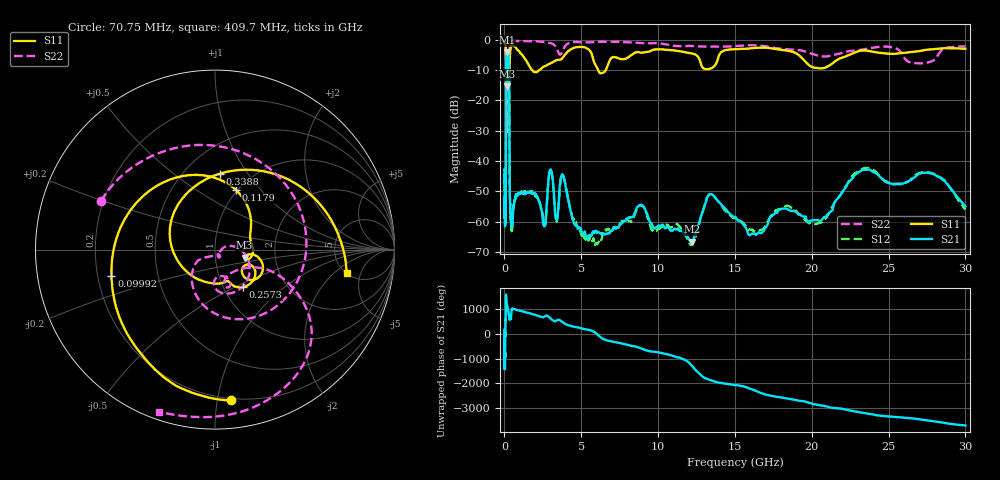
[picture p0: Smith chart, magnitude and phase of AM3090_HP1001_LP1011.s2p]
! Date/Time: Thu, Feb 28, 2019 2:03 PM
! Network Analyzer: Agilent Technologies E8364B Rev: A.07.50.67
! Sweep from 0.010 to 30.000 GHz, 1601 Points, Sweep Type: LOG
! Power Supply: 5.022 V, 0.002 A
# Hz S DB R 50
!freq MagS11 AngS11 MagS21 AngS21 MagS12 AngS12 MagS22 AngS22
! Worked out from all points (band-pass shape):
!   1601 points, 10 MHz to 30 GHz, reference 50 ohm
!   highest |S21| = -4.03 dB at 170.7 MHz (marker M1); lowest = -66.7 dB at 12.19 GHz (marker M2)
!   |S21| within 3 dB of the highest: 124.9 MHz to 287.7 MHz (162.7 MHz wide, 78.9 % of centre)
!   lowest |S11| = -15.3 dB at 154.4 MHz (marker M3), VSWR 1.41, Z = 69.4 - j6.43 ohm
!   |S11| at or under -10 dB: 119.6 MHz to 326.2 MHz (206.6 MHz wide, 92.7 % of centre); 1.812 GHz to 2.24 GHz (427.5 MHz wide, 21.1 % of centre); 6.098 GHz to 6.588 GHz (490 MHz wide, 7.72 % of centre)
!   |S22| runs from -30.9 to -0.2 dB; largest |S21 - S12| = 0.011
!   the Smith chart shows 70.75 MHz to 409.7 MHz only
!   S11 on the Smith chart (normalised r, x): 70.75 MHz: 0.19, -1.10; 99.92 MHz: 0.26, -0.12; 117.9 MHz: 0.98, +0.75; 257.3 MHz: 1.24, -0.55; 338.8 MHz: 0.73, +0.75; 409.7 MHz: 5.09, -2.92
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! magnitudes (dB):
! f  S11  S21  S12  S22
! 10 MHz  -0.3  -42.9  -45.6  -0.6
! 38.04 MHz  -0.5  -59.7  -59.0  -1.6
! 70.75 MHz  -1.5  -56.0  -52.0  -3.2
! 99.92 MHz  -4.5  -35.5  -36.0  -5.7
! 117.9 MHz  -9.1  -11.3  -11.3  -11.3
! 144.7 MHz  -14.1  -4.5  -4.5  -30.6
! 154.4 MHz  -15.3  -4.2  -4.2  -25.4
! 170.7 MHz  -12.7  -4.0  -4.0  -14.3
! 257.3 MHz  -11.7  -4.9  -4.9  -13.0
! 300.5 MHz  -14.5  -10.2  -10.1  -10.1
! 338.8 MHz  -7.5  -44.8  -44.8  -1.3
! 409.7 MHz  -2.6  -58.7  -59.0  -0.4
! 550.5 MHz  -1.9  -57.1  -57.7  -0.3
! 2.084 GHz  -10.6  -51.5  -51.5  -0.5
! 2.597 GHz  -8.7  -61.3  -61.4  -0.6
! 3.002 GHz  -7.7  -42.8  -42.9  -1.1
! 7.926 GHz  -6.1  -59.6  -59.1  -0.7
! 12.19 GHz  -4.4  -66.7  -67.8  -2.0
! 13.54 GHz  -9.1  -51.1  -51.3  -2.2
! 20.31 GHz  -9.2  -59.6  -60.8  -5.0
! 23.48 GHz  -3.5  -42.9  -42.3  -3.0
! 30 GHz  -2.9  -55.0  -56.1  -2.1
